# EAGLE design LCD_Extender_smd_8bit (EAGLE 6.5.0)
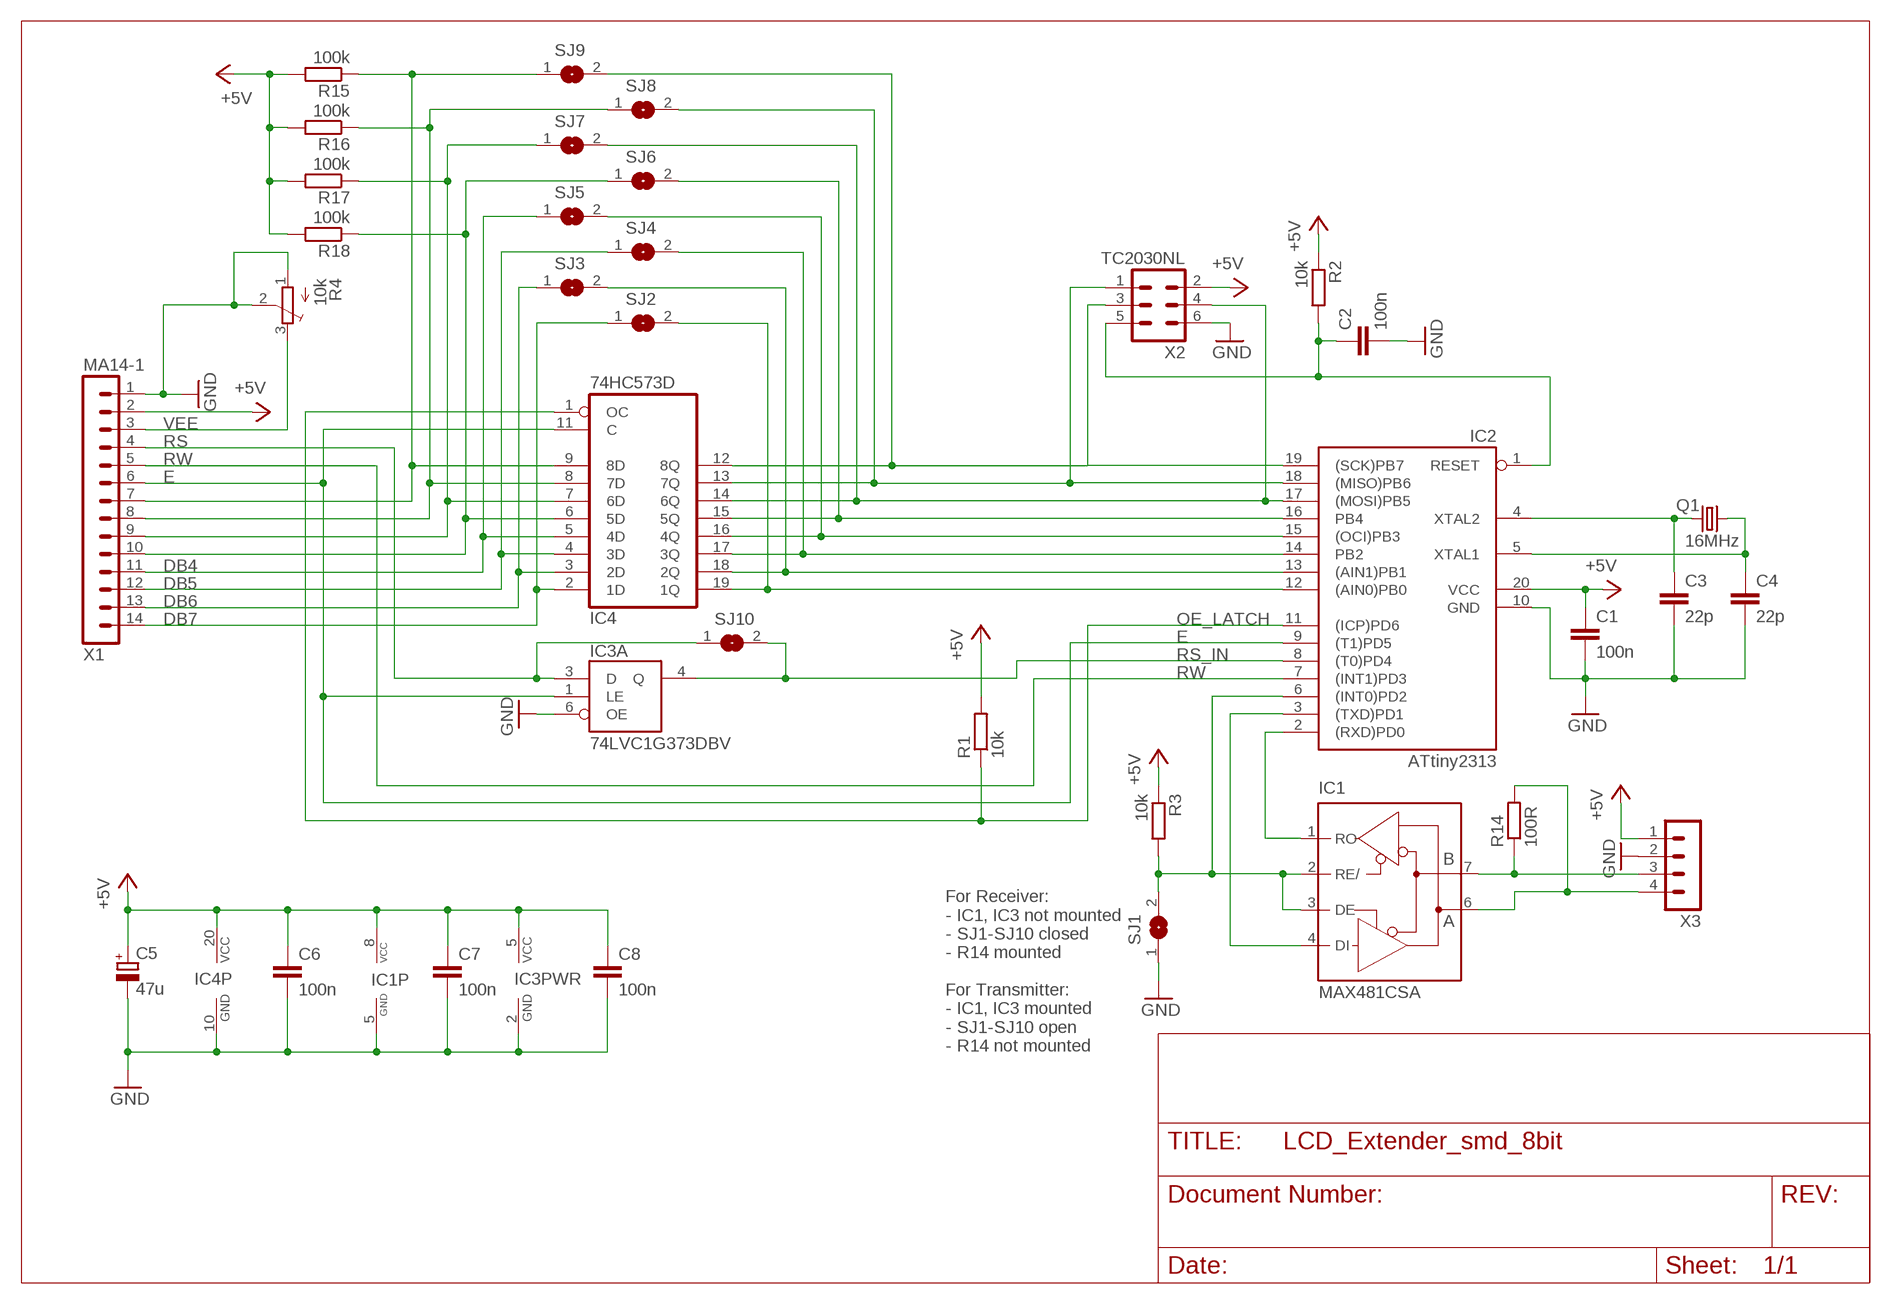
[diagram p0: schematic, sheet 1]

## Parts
C1  100n  C-EUC1206  [C1206]
C2  100n  C-EUC1206  [C1206]
C3  22p  C-EUC1206  [C1206]
C4  22p  C-EUC1206  [C1206]
C5  47u  CPOL-EUCT3528  [CT3528]
C6  100n  C-EUC1206  [C1206]
C7  100n  C-EUC1206  [C1206]
C8  100n  C-EUC1206  [C1206]
IC1  MAX481CSA  [SO08]
IC2  ATtiny2313  AT90S2313S  [SO20L]
IC3  74LVC1G373DBV  [SOT23-6]
IC4  74HC573D  [SO20W]
Q1  16MHz  CRYSTALHC49UP  [HC49UP]
R1  10k  R-EU_R1206  [R1206]
R2  10k  R-EU_R1206  [R1206]
R3  10k  R-EU_R1206  [R1206]
R4  10k  TRIM_EU-3223G  [3223G]
R14  100R  R-EU_R1206  [R1206]
R15  100k  R-EU_R1206  [R1206]
R16  100k  R-EU_R1206  [R1206]
R17  100k  R-EU_R1206  [R1206]
R18  100k  R-EU_R1206  [R1206]
SJ1  SJ  [SJ]
SJ2  SJ0603  [SJ0603]
SJ3  SJ0603  [SJ0603]
SJ4  SJ0603  [SJ0603]
SJ5  SJ0603  [SJ0603]
SJ6  SJ0603  [SJ0603]
SJ7  SJ0603  [SJ0603]
SJ8  SJ0603  [SJ0603]
SJ9  SJ0603  [SJ0603]
SJ10  SJ0603  [SJ0603]
X1  MA14-1  [MA14-1]
X2  TC2030NL  [TC2030-IDC-NL]
X3  MA04-1  [MA04-1]

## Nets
+5V: C1.1 C5.+ C6.1 C7.1 C8.1 IC1.8(VCC) IC2.20(VCC) IC3.5(PWR:VCC) IC4.20(VCC) R1.2 R2.1 R3.1 R15.2 R16.2 R17.2 R18.2 X1.2 X2.2 X3.1
DB4: IC4.5(4D) SJ5.1 X1.11
DB5: IC4.4(3D) SJ4.1 X1.12
DB6: IC4.3(2D) SJ3.1 X1.13
DB7: IC4.2(1D) SJ2.1 X1.14
E: IC2.9((T1)PD5) IC3.1(A:LE) IC4.11(C) X1.6
GND: C1.2 C2.2 C3.2 C4.2 C5.- C6.2 C7.2 C8.2 IC1.5(GND) IC2.10(GND) IC3.2(PWR:GND) IC3.6(A:OE) IC4.10(GND) R4.1(A) R4.2(S) SJ1.1 X1.1 X2.6 X3.2
N$1: IC2.17((MOSI)PB5) IC4.14(6Q) SJ7.2 X2.4
N$2: C3.1 IC2.4(XTAL2) Q1.1
N$3: IC2.15((OCI)PB3) IC4.16(4Q) SJ5.2
N$4: IC2.16(PB4) IC4.15(5Q) SJ6.2
N$5: IC2.18((MISO)PB6) IC4.13(7Q) SJ8.2 X2.1
N$7: IC1.4(DI) IC2.3((TXD)PD1)
N$8: IC4.7(6D) R17.1 SJ7.1 X1.9
N$9: C4.1 IC2.5(XTAL1) Q1.2
N$10: IC1.7(B) R14.1 X3.3
N$13: IC4.8(7D) R16.1 SJ8.1 X1.8
N$14: C2.1 IC2.1(RESET) R2.2 X2.5
N$17: IC4.6(5D) R18.1 SJ6.1 X1.10
N$18: IC4.9(8D) R15.1 SJ9.1 X1.7
N$19: IC1.6(A) R14.2 X3.4
N$23: IC2.19((SCK)PB7) IC4.12(8Q) SJ9.2 X2.3
N$25: IC2.12((AIN0)PB0) IC4.19(1Q) SJ2.2
N$26: IC2.13((AIN1)PB1) IC4.18(2Q) SJ3.2
N$27: IC2.14(PB2) IC4.17(3Q) SJ4.2
N$29: IC1.1(RO) IC2.2((RXD)PD0)
N$30: IC1.2(RE/) IC1.3(DE) IC2.6((INT0)PD2) R3.2 SJ1.2
OE_LATCH: IC2.11((ICP)PD6) IC4.1(OC) R1.1
RS: IC3.3(A:D) SJ10.1 X1.4
RS_IN: IC2.8((T0)PD4) IC3.4(A:Q) SJ10.2
RW: IC2.7((INT1)PD3) X1.5
VEE: R4.3(E) X1.3

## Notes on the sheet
- For Receiver:
  - IC1, IC3 not mounted
  - SJ1-SJ10 closed
  - R14 mounted
  
  For Transmitter:
  - IC1, IC3 mounted
  - SJ1-SJ10 open
  - R14 not mounted

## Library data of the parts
C1-C4 C6-C8 = rcl:C-EU: CAPACITOR, European symbol
C5 = rcl:CPOL-EU: POLARIZED CAPACITOR, European symbol
IC1 = maxim:MAX481CSA: RS485 TRANSEIVER; MF: MAXIM; MPN: MAX481CSA; OC_FARNELL: unknown; OC_NEWARK: 90C3817
IC2 = atmel:AT90S2313: MICROCONTROLLER 2 Kbytes FLASH 128 bytes SRAM 128 bytes EEPROM UART; OC_FARNELL: unknown; OC_NEWARK: unknown
IC3 = Brunner:74LVC1G373
IC4 = 74xx-eu:74*573: 8-bit D latch BUS DRIVER
Q1 = crystal:CRYSTAL: CRYSTAL; OC_FARNELL: unknown; OC_NEWARK: unknown
R1-R3 R14-R18 = rcl:R-EU_: RESISTOR, European symbol
R4 = pot:TRIM_EU-: POTENTIOMETER
SJ1 = jumper:SJ: SMD solder JUMPER
SJ2-SJ10 = Brunner:SJ: SMD solder JUMPER
X1 = Brunner:MA14-1
X2 = Brunner:TC2030
X3 = con-lstb:MA04-1: PIN HEADER; OC_FARNELL: unknown; OC_NEWARK: unknown

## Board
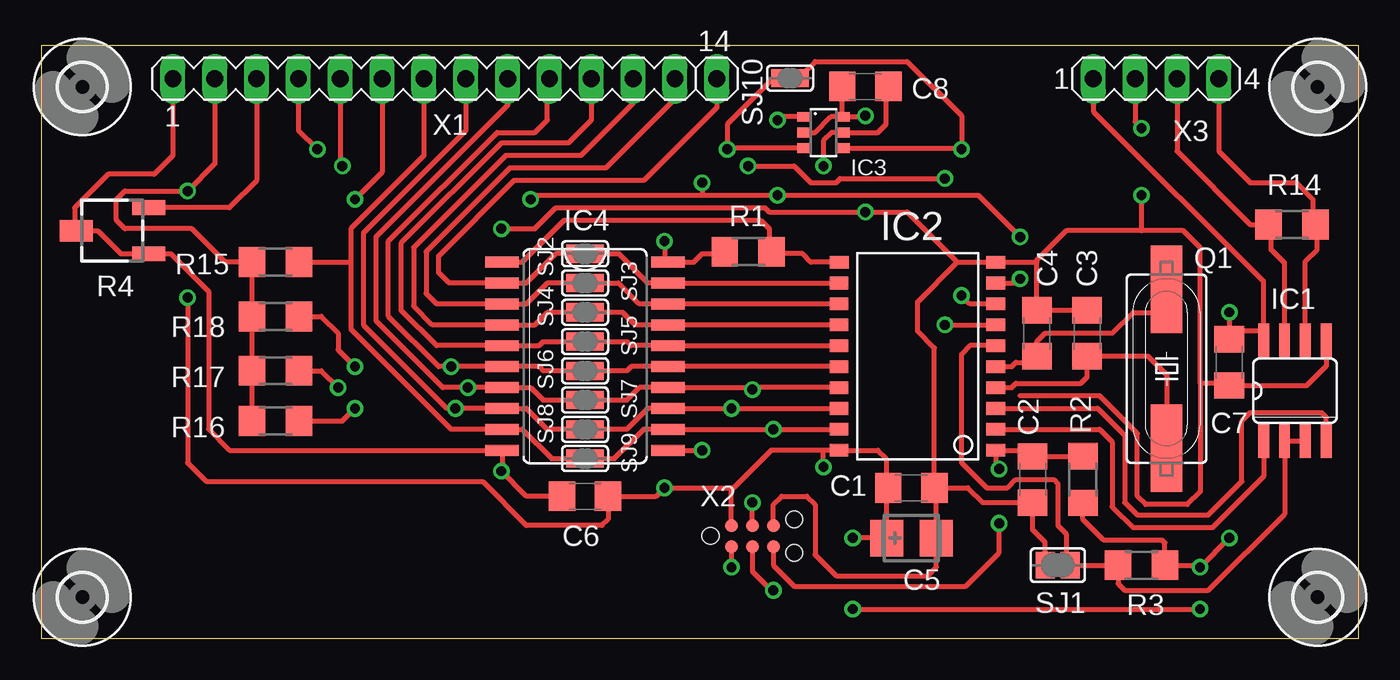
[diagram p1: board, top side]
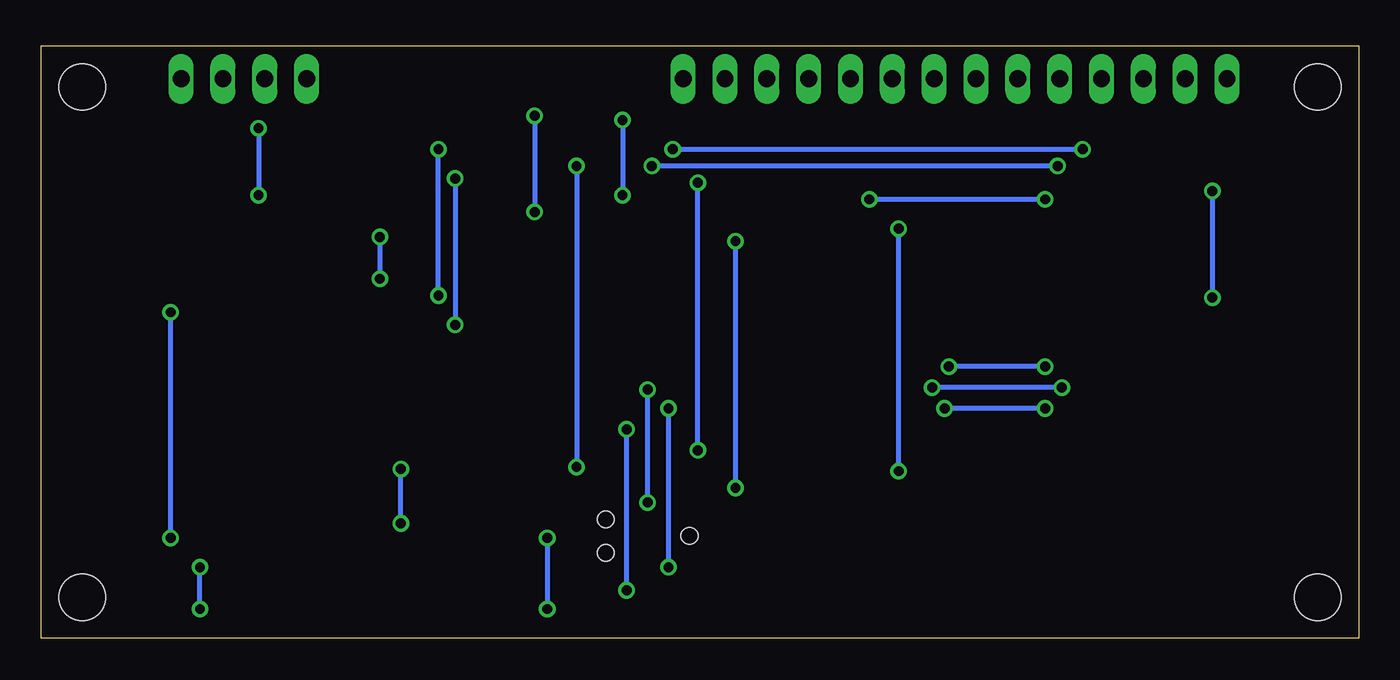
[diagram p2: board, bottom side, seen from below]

Size 80 x 36 mm. Coordinates in mm from the lower left corner, seen from the top.
Outline: 0,36 0,0 80,0 80,36 0,36
Copper layers (1*16): Top 0.035mm / dielectric 1.5mm / Bottom 0.035mm
Design rules "default *": minimum track width 10mil, minimum drill 0.6mm, track to track 0.3mm, track to pad 0.3mm, pad to pad 0.3mm, via to via 0.3mm, smd to smd 8mil, copper to edge 0.4mm, drill to drill 8mil, minimum pad ring 10mil, minimum via ring 8mil, stop-mask expansion 4mil, vias tented up to drill 0mil, thermal gap 10mil

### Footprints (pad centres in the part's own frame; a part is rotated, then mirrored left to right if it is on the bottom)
C1206 = smd 1.6 x 1.8: 1 -1.4,0; 2 1.4,0
CT3528 = smd 2 x 2.2: + -1.5,0; - 1.5,0
SO08 = smd 0.66 x 2.032: 1 -1.905,-3.073; 2 -0.635,-3.073; 3 0.635,-3.073; 4 1.905,-3.073; 5 1.905,3.073; 6 0.635,3.073; 7 -0.635,3.073; 8 -1.905,3.073
SO20L = smd 0.762 x 1.143: 1 -5.08,-5.131; 2 -3.81,-5.131; 3 -2.54,-5.131; 4 -1.27,-5.131; 5 0,-5.131; 6 1.27,-5.131; 7 2.54,-5.131; 8 3.81,-5.131; 9 5.08,-5.131; 10 6.35,-5.131; 11 6.35,4.369; 12 5.08,4.394; 13 3.81,4.394; 14 2.54,4.394; 15 1.27,4.394; 16 0,4.394; 17 -1.27,4.394; 18 -2.54,4.394; 19 -3.81,4.394; 20 -5.08,4.394
SOT23-6 = smd 0.6 x 0.9: 1 -0.95,-1.15; 2 0,-1.15; 3 0.95,-1.15; 4 0.95,1.15; 5 0,1.15; 6 -0.95,1.15
SO20W = smd 0.66 x 2.032: 1 -5.715,-5.029; 2 -4.445,-5.029; 3 -3.175,-5.029; 4 -1.905,-5.029; 5 -0.635,-5.029; 6 0.635,-5.029; 7 1.905,-5.029; 8 3.175,-5.029; 9 4.445,-5.029; 10 5.715,-5.029; 11 5.715,5.029; 12 4.445,5.029; 13 3.175,5.029; 14 1.905,5.029; 15 0.635,5.029; 16 -0.635,5.029; 17 -1.905,5.029; 18 -3.175,5.029; 19 -4.445,5.029; 20 -5.715,5.029
HC49UP = smd 5.334 x 1.93: 1 -4.826,0; 2 4.826,0
R1206 = smd 1.6 x 1.803: 1 -1.422,0; 2 1.422,0
3223G = smd 2 x 0.9: 1 -2.2,1.4; 3 -2.2,-1.4 | smd 2 x 1.3: 2 2.2,0
SJ = smd 1.168 x 1.6: 1 -0.762,0; 2 0.762,0
SJ0603 = smd 1 x 1.1: 1 -0.635,0; 2 0.635,0
2,8 = hole 2.8: 0,0
MA14-1 = drill 1.016 long: 1 -16.51,0; 2 -13.97,0; 3 -11.43,0; 4 -8.89,0; 5 -6.35,0; 6 -3.81,0; 7 -1.27,0; 8 1.27,0; 9 3.81,0; 10 6.35,0; 11 8.89,0; 12 11.43,0; 13 13.97,0; 14 16.51,0
TC2030-IDC-NL = smd 0.78 x 0.78: 1 -1.27,-0.635; 2 -1.27,0.635; 3 0,-0.635; 4 0,0.635; 5 1.27,-0.635; 6 1.27,0.635 | hole 1: -2.54,0; 2.54,1.016; 2.54,-1.016
MA04-1 = drill 1.016 long: 1 -3.81,0; 2 -1.27,0; 3 1.27,0; 4 3.81,0

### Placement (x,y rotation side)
C1  52.83,9.14 0 top
C2  60.2,9.65 270 top
C3  63.5,18.54 90 top
C4  60.45,18.54 90 top
C5  52.83,6.1 0 top
C6  33.02,8.64 180 top
C7  72.14,16.76 270 top
C8  50.04,33.53 180 top
IC1  76.12,15.04 0 top
IC2  52.83,16.51 90 top
IC3  47.5,30.73 270 top
IC4  33.02,17.14 270 top
Q1  68.33,16.38 90 top
R1  42.93,23.5 180 top
R2  63.25,9.65 90 top
R3  66.8,4.45 180 top
R4  4.32,24.77 180 top
R14  75.95,25.15 0 top
R15  14.22,22.86 180 top
R16  14.22,13.21 180 top
R17  14.22,16.26 180 top
R18  14.22,19.56 180 top
SJ1  61.72,4.45 0 top
SJ2  33.02,23.37 0 top
SJ3  33.02,21.59 0 top
SJ4  33.02,19.81 0 top
SJ5  33.02,18.03 0 top
SJ6  33.02,16.26 0 top
SJ7  33.02,14.48 0 top
SJ8  33.02,12.7 0 top
SJ9  33.02,10.92 0 top
SJ10  45.47,34.04 0 top
U$1  [2,8]  2.5,33.5 0 top
U$2  [2,8]  2.5,2.5 0 top
U$3  [2,8]  77.5,2.5 0 top
U$4  [2,8]  77.5,33.5 0 top
X1  24.51,34 0 top
X2  43.18,6.22 0 top
X3  67.69,34 0 top

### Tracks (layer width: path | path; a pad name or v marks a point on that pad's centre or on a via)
+5V  (via drill 0.6)
  Top 0.305: 41.91,9.14 v37.85,9.14 37.34,8.64 C6.1 34.42,7.24 34.04,6.86 29.46,6.86 26.8,9.53 10.03,9.53 8.89,10.67 v8.89,20.7 | 41.91,9.14 42.04,9.14 44.32,11.43 47.5,11.43 | 47.5,11.43 IC2.20 50.8,11.43 51.31,10.92 51.31,9.27 C1.1 51.33,9.04 C5.+ v49.28,6.1 | 63.25,8.48 R2.1 63.25,7.24 64.52,5.97 68.07,5.97 68.22,5.82 R3.1 70.23,4.45 v70.36,4.32 v72.14,6.1 | v72.14,19.81 C7.1 72.64,18.67 74.17,18.67 74.22,18.62 IC1.8 74.22,21.67 63.88,32 X3.1 | X2.2 41.91,9.14 | R1.2 41.38,23.37 40.13,23.37 39.62,22.86 IC4.20 37.85,23.06 v37.85,24.13 | X1.2 10.54,28.83 v8.89,27.18 5.08,27.18 4.57,26.67 4.57,25.4 5.08,24.89 9.14,24.89 11.18,22.86 R15.2 R18.2 R17.2 R16.2 | v49.28,1.78 v70.36,1.78 | C8.1 51.31,33.4 51.31,31.24 50.8,30.73 IC3.5 48.01,30.73 47.5,30.23 v47.5,28.7 | v47.5,10.41 47.5,11.43
  Bottom 0.305: v37.85,24.13 v37.85,9.14 | v8.89,27.18 v8.89,20.7 | v49.28,6.1 v49.28,1.78 | v70.36,1.78 v70.36,4.32 | v72.14,6.1 v72.14,19.81 | v47.5,28.7 v47.5,10.41
DB4
  Top 0.305: X1.11 33.4,31.5 32,30.1 27.94,30.1 21.84,24 21.84,19.94 24,17.78 IC4.5 30.23,17.78 30.48,18.03 SJ5.1
DB5
  Top 0.305: X1.12 35.94,32.51 32.77,29.34 28.19,29.34 22.61,23.75 22.61,20.19 23.75,19.05 IC4.4 29.97,19.05 30.73,19.81 SJ4.1
DB6
  Top 0.305: X1.13 38.48,32.77 34.29,28.57 28.45,28.57 23.37,23.5 23.37,20.95 24,20.32 IC4.3 29.46,20.32 30.73,21.59 SJ3.1
DB7
  Top 0.305: X1.14 41.02,32.26 36.58,27.81 28.7,27.81 24.13,23.24 24.13,22.23 24.77,21.59 IC4.2 29.46,21.59 31.24,23.37 SJ2.1
E  (via drill 0.6)
  Top 0.305: v29.72,26.67 29.97,26.92 40.13,26.92 | 40.13,26.92 v44.7,26.92 56.9,26.92 v59.44,24.38 | IC2.9 59.18,21.59 v59.44,21.84 | IC4.11 v40.13,11.43 | v40.13,27.69 40.13,26.92 | X1.6 20.7,28.32 v19.05,26.67 | IC3.1 44.89,31.68 v44.7,31.5
  Bottom 0.305: v19.05,26.67 v29.72,26.67 | v59.44,24.38 v59.44,21.84 | v40.13,11.43 v40.13,27.69 | v44.7,31.5 v44.7,26.92
GND  (via drill 0.6)
  Top 0.305: 55.63,22.86 53.22,20.45 53.22,18.67 54.23,17.65 C1.2 | 55.63,22.86 IC2.10 60.45,22.86 | C3.2 C4.2 60.45,22.86 | C1.2 56.26,9.14 57.15,8.25 C2.2 60.2,6.6 60.96,5.84 SJ1.1 | 55.63,22.86 52.58,25.91 v50.04,25.91 44.2,25.91 43.94,26.16 31.24,26.16 29.97,24.89 v27.94,24.89 | 66.8,24.77 69.34,24.77 70.36,23.75 70.36,15.49 | 66.8,24.77 62.23,24.77 60.45,22.99 60.45,22.86 | X1.1 8,29.34 6.86,28.19 4.06,28.19 2.03,26.16 2.03,24.85 R4.2 3.43,24.77 4.83,23.37 R4.1 7.88,23.36 10.16,21.08 10.16,12.7 11.43,11.43 IC4.10 27.99,10.21 v27.94,10.16 29.46,8.64 C6.2 | 59.44,14.73 64.26,14.73 66.55,12.45 66.55,8.64 67.06,8.13 69.6,8.13 70.36,8.89 70.36,15.49 | IC1.5 78.03,16.56 76.83,15.36 C7.2 72.01,15.49 70.36,15.49 | X3.2 66.42,31.37 v66.8,30.99 | v66.8,26.92 66.8,24.77 | X2.6 44.45,8.13 44.96,8.64 46.48,8.64 46.99,8.13 46.99,5.08 48.26,3.81 53.85,3.81 54.36,4.32 54.36,6.07 C5.- 54.33,9.04 C1.2 | IC3.2 46.99,30.73 47.94,31.68 IC3.6 | IC3.6 49.97,31.68 v50.04,31.75 | IC3.6 48.65,33.52 C8.2
  Bottom 0.305: v27.94,10.16 v27.94,24.89 | v66.8,30.99 v66.8,26.92 | v50.04,31.75 v50.04,25.91
N$1  (via drill 0.6)
  Top 0.305: X2.4 v43.18,8.26 | IC2.17 43.31,15.24 v43.18,15.11 43.05,15.24 IC4.14 36.32,15.24 35.56,14.48 SJ7.2
  Bottom 0.305: v43.18,8.26 v43.18,15.11
N$2
  Top 0.305: IC2.4 58.93,15.24 59.18,15.49 63.12,15.49 63.5,15.88 C3.1 67.19,17.14 68.33,16 Q1.1
N$3
  Top 0.305: IC2.15 IC4.16 35.81,17.78 35.56,18.03 SJ5.2
N$4
  Top 0.305: IC2.16 IC4.15 35.81,16.51 35.56,16.26 SJ6.2
N$5  (via drill 0.6)
  Top 0.305: X2.1 v41.91,4.32 | IC2.18 v41.91,13.97 IC4.13 36.83,13.97 35.56,12.7 SJ8.2
  Bottom 0.305: v41.91,4.32 v41.91,13.97
N$7
  Top 0.305: IC2.3 64.14,13.97 65.79,12.32 65.79,8.26 66.55,7.49 70.87,7.49 72.9,9.53 72.9,13.21 73.41,13.72 77.72,13.72 78.03,13.41 IC1.4
N$8  (via drill 0.6)
  Top 0.305: X1.9 28.32,32.38 20.32,24.38 20.32,19.3 24.38,15.24 v25.91,15.24 IC4.7 29.72,15.24 30.48,14.48 SJ7.1 | R17.1 17.02,16.26 v18.03,15.24
  Bottom 0.305: v18.03,15.24 v25.91,15.24
N$9
  Top 0.305: Q1.2 68.33,20.32 67.82,19.81 66.29,19.81 65.02,18.54 60.96,18.54 60.45,18.03 C4.1 60.07,16.76 59.18,16.76 58.93,16.51 IC2.5
N$10
  Top 0.305: IC1.7 75.49,22.81 74.68,23.62 74.68,24.99 R14.1 73.41,25.15 68.96,29.59 X3.3
N$13  (via drill 0.6)
  Top 0.305: X1.8 25.78,30.86 19.56,24.64 19.56,19.05 24.64,13.97 v25.15,13.97 IC4.8 29.46,13.97 30.73,12.7 SJ8.1 | R16.1 18.29,13.21 v19.05,13.97
  Bottom 0.305: v19.05,13.97 v25.15,13.97
N$14  (via drill 0.6)
  Top 0.305: X2.5 44.45,4.45 45.72,3.17 56.13,3.17 58.17,5.21 v58.17,6.99 | v58.17,10.29 57.96,10.49 IC2.1 59.82,11.43 C2.1 63.22,11.05 R2.2
  Bottom 0.305: v58.17,6.99 v58.17,10.29
N$17  (via drill 0.6)
  Top 0.305: X1.10 30.73,33.87 30.73,31.5 29.97,30.73 27.69,30.73 21.08,24.13 21.08,19.56 24.13,16.51 v24.89,16.51 IC4.6 30.23,16.51 30.48,16.26 SJ6.1 | R18.1 17.02,19.56 18.03,18.54 18.03,17.53 v19.05,16.51
  Bottom 0.305: v19.05,16.51 v24.89,16.51
N$18
  Top 0.305: X1.7 23.24,29.34 18.8,24.89 18.8,22.86 | 18.8,22.86 18.8,18.8 24.89,12.7 IC4.9 29.21,12.7 30.99,10.92 SJ9.1 | R15.1 18.8,22.86
N$19
  Top 0.305: IC1.6 76.76,22.91 77.47,23.62 77.47,25.04 R14.2 77.22,25.3 77.22,26.67 76.2,27.69 73.41,27.69 71.5,29.59 X3.4
N$23  (via drill 0.6)
  Top 0.305: X2.3 43.18,4.06 44.32,2.92 v44.45,2.92 | IC2.19 v44.45,12.7 IC4.12 36.58,12.7 34.8,10.92 SJ9.2
  Bottom 0.305: v44.45,2.92 v44.45,12.7
N$25
  Top 0.305: IC2.12 IC4.19 36.83,21.59 35.05,23.37 SJ2.2
N$26
  Top 0.305: IC2.13 IC4.18 36.32,20.32 35.05,21.59 SJ3.2
N$27
  Top 0.305: IC2.14 IC4.17 36.07,19.05 35.31,19.81 SJ4.2
N$29
  Top 0.305: IC1.1 74.22,9.83 71.12,6.73 66.29,6.73 65.02,8 65.02,11.94 64.26,12.7 IC2.2
N$30
  Top 0.305: IC1.3 IC1.2 75.49,7.54 70.87,2.92 65.79,2.92 65.38,3.33 R3.2 SJ1.2 62.23,4.7 62.23,6.35 61.72,6.86 61.72,9.4 61.47,9.65 59.18,9.65 58.67,9.14 57.4,9.14 55.88,10.67 55.88,17.27 56.39,17.78 IC2.6
OE_LATCH
  Top 0.305: IC4.1 29.21,22.86 31.75,25.4 43.69,25.4 44.2,24.89 44.2,23.65 R1.1 44.48,23.37 46.23,23.37 46.74,22.86 IC2.11
RS  (via drill 0.6)
  Top 0.305: v16.76,29.72 15.62,30.86 X1.4 | IC3.3 41.72,29.78 v41.66,29.72 41.66,31.24 44.45,34.04 SJ10.1
  Bottom 0.305: v41.66,29.72 v16.76,29.72
RS_IN  (via drill 0.6)
  Top 0.305: IC2.8 56.39,20.32 v55.88,20.83 | IC3.4 55.81,29.78 v55.88,29.72 55.88,31.75 52.58,35.05 46.99,35.05 46.1,34.16 SJ10.2
  Bottom 0.305: v55.88,20.83 v55.88,29.72
RW  (via drill 0.6)
  Top 0.305: X1.5 18.16,28.83 v18.29,28.7 | v42.93,28.7 45.72,28.7 46.74,27.69 48.26,27.69 48.51,27.94 v54.86,27.94 | v54.86,19.05 IC2.7
  Bottom 0.305: v18.29,28.7 v42.93,28.7 | v54.86,27.94 v54.86,19.05
VEE
  Top 0.305: X1.3 13.08,27.81 11.43,26.16 R4.3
